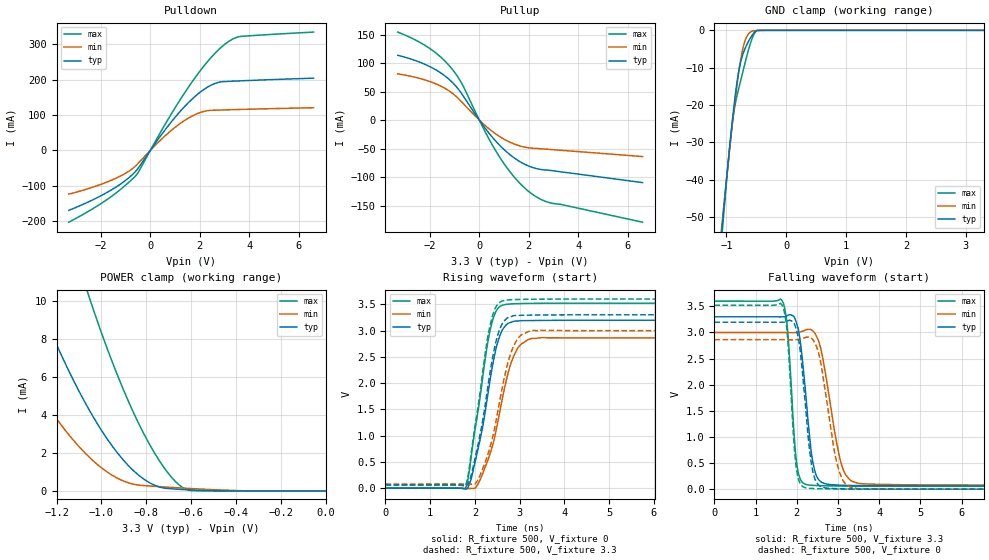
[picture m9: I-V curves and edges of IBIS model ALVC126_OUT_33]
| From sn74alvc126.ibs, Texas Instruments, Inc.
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[Model]   ALVC126_OUT_33
Model_type  3-state
Enable   Active-High
Vref =   0
Rref =   500
Cref =   50p
Vmeas =   1.5
| variable   typ   min   max
C_comp   4.92pF   4.23pF   5.84pF
| C_pullup   6.06pF   4.27pF   7.77pF
| C_pulldown   7.87pF   4.86pF   12.41pF
| C_tri-state   4.92pF   4.23pF   5.84pF
[Temperature Range]   40   100   -40
| Ambient temperature   25   85   -40
[Voltage range]   3.3   3   3.6
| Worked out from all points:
|   slope of the pulldown table from 0 to 0.495 V, typ, clamps not added: 10.2 ohm
|   slope of the pullup table from 0 to 0.495 V, typ, clamps not added: 17.4 ohm
|   GND clamp passes 1 mA (typ) near -0.56 V on its own axis
|   POWER clamp passes 1 mA (typ) near -0.85 V on its own axis
|   rising waveform, R_fixture 500, V_fixture 0: 20-80 % time 405ps typ, 469ps min, 364ps max; typ from 0 V to 3.2 V
|   falling waveform, R_fixture 500, V_fixture 3.3: 20-80 % time 240ps typ, 374ps min, 169ps max; typ from 3.3 V to 0.064 V
|   rising waveform, R_fixture 500, V_fixture 3.3: 20-80 % time 395ps typ, 450ps min, 358ps max; typ from 0.064 V to 3.3 V
|   falling waveform, R_fixture 500, V_fixture 0: 20-80 % time 232ps typ, 343ps min, 164ps max; typ from 3.2 V to 0 V
[GND Clamp]
| ALVC126_OUT_33
|   Voltage   I(typ)   I(min)   I(max)
-3.3V     -502.3mA   -462.6mA   -544.6mA
-1.08V    -54.25mA   -52.87mA   -55.93mA
-1.06V    -50.69mA   -49.62mA   -52.05mA
-965mV    -34.4mA    -34.63mA   -34.59mA
-900mV    -24.12mA   -24.99mA   -24.7mA
-860mV    -18.44mA   -19.43mA   -20.39mA
-805mV    -11.98mA   -12.5mA    -16.29mA
-705mV    -5.559mA   -3.602mA   -9.787mA
-655mV    -3.719mA   -1.531mA   -6.626mA
-575mV    -1.408mA   -240.7uA   -2.39mA
-480mV    -21.04uA   -62.18uA   -16.51uA
3.3V      104.8pA    1.494uA    43.91pA
[POWER Clamp]
| ALVC126_OUT_33
|   Voltage   I(typ)   I(min)   I(max)
-3.3V     101.4mA    70.85mA    144.9mA
-1.515V   17.49mA    10.21mA    30.43mA
-1.39V    13.28mA    7.381mA    24.27mA
-1.295V   10.36mA    5.473mA    19.9mA
-1.175V   7.064mA    3.406mA    14.79mA
-1.055V   4.279mA    1.788mA    10.22mA
-950mV    2.335mA    812.2uA    6.743mA
-845mV    938.6uA    325.5uA    3.823mA
-745mV    219.5uA    228.1uA    1.65mA
-655mV    86.61uA    162.8uA    329uA
-600mV    50.74uA    125.6uA    17.36uA
-48.03fV  104.8pA    414.1pA    48.4pA
[Pulldown]
| ALVC126_OUT_33
|   Voltage   I(typ)   I(min)   I(max)
-3.3V     -169.5mA   -123.9mA   -203mA
-1.625V   -113.8mA   -85.92mA   -132.9mA
-1.02V    -85.87mA   -65.43mA   -99.42mA
-590mV    -58.76mA   -43.67mA   -71.86mA
600mV     58.25mA    41.24mA    73.83mA
1.525V    133.8mA    90.44mA    177mA
2.34V     179.7mA    112.3mA    253mA
2.695V    190.8mA    113.5mA    279.9mA
3.025V    194.3mA    114.3mA    300.3mA
3.355V    195.4mA    114.9mA    315.1mA
3.65V     196.3mA    115.5mA    321.7mA
6.6V      203.8mA    120.3mA    334mA
[Pullup]
| ALVC126_OUT_33
|   Voltage   I(typ)   I(min)   I(max)
-3.3V     113.7mA    81.1mA     154.3mA
-2.045V   94.71mA    68.29mA    126.7mA
-1.555V   82.58mA    59.54mA    110.3mA
-1.135V   67.94mA    48.5mA     91.26mA
-685mV    44.37mA    30.46mA    62.31mA
200mV     -12.17mA   -8.178mA   -17.55mA
785mV     -42.51mA   -27.85mA   -62.43mA
1.415V    -66.5mA    -42.01mA   -100.1mA
2.045V    -81.49mA   -48.91mA   -126.8mA
2.445V    -86.35mA   -50.12mA   -138.1mA
2.85V     -88.18mA   -51.47mA   -145mA
6.6V      -109.6mA   -63.97mA   -179.1mA
[Ramp]
| ALVC126_OUT_33
| variable   typ   min   max
dV/dt_r   1.93/4.10E-10   1.72/4.78E-10   2.12/3.68E-10
dV/dt_f   1.97/2.53E-10   1.79/3.89E-10   2.15/1.78E-10
R_load = 500
[Rising Waveform]
| ALVC126_OUT_33
R_fixture =   500
C_fixture =   0
L_fixture =   0
V_fixture =   0
V_fixture_min = 0
V_fixture_max = 0
|   Time   V(typ)   V(min)   V(max)
0s        33.51pV    1.907nV    27.94pV
1.78ns    -11.41mV   -1.75mV    -14.61mV
1.945ns   280.2mV    -4.234mV   783.1mV
2.18ns    1.202V     293.1mV    2.158V
2.35ns    2.124V     689.7mV    3.048V
2.53ns    2.838V     1.345V     3.438V
2.725ns   3.128V     2.139V     3.503V
3.01ns    3.187V     2.724V     3.514V
3.52ns    3.194V     2.866V     3.52V
50ns      3.197V     2.862V     3.521V
[Falling Waveform]
| ALVC126_OUT_33
R_fixture =   500
C_fixture =   0
L_fixture =   0
V_fixture =   3.3
V_fixture_min = 3
V_fixture_max = 3.6
|   Time   V(typ)   V(min)   V(max)
0s        3.3V       3V         3.6V
1.655ns   3.3V       3V         3.592V
1.775ns   3.324V     2.999V     3.055V
2.005ns   3.154V     3V         452.2mV
2.12ns    2.596V     3.02V      147.2mV
2.33ns    863.9mV    3.058V     75.48mV
2.585ns   140mV      2.683V     67.18mV
3.11ns    74.4mV     410.1mV    58.46mV
3.645ns   66.34mV    100.5mV    56.19mV
50ns      63.7mV     79.91mV    56.01mV
[Rising Waveform]
| ALVC126_OUT_33
R_fixture =   500
C_fixture =   0
L_fixture =   0
V_fixture =   3.3
V_fixture_min = 3
V_fixture_max = 3.6
|   Time   V(typ)   V(min)   V(max)
0s        63.7mV     79.91mV    56.01mV
1.78ns    52.24mV    77.86mV    41.44mV
1.86ns    108.8mV    74.8mV     311.8mV
2ns       561.6mV    79.22mV    1.179V
2.34ns    2.221V     791.9mV    3.108V
2.52ns    2.945V     1.504V     3.514V
2.72ns    3.238V     2.334V     3.582V
3.005ns   3.291V     2.894V     3.593V
3.515ns   3.297V     3.006V     3.599V
50ns      3.3V       3V         3.6V
[Falling Waveform]
| ALVC126_OUT_33
R_fixture =   500
C_fixture =   0
L_fixture =   0
V_fixture =   0
V_fixture_min = 0
V_fixture_max = 0
|   Time   V(typ)   V(min)   V(max)
0s        3.197V     2.862V     3.521V
1.65ns    3.197V     2.862V     3.512V
1.765ns   3.216V     2.861V     3.01V
1.99ns    3.054V     2.862V     395.2mV
2.1ns     2.528V     2.877V     83.95mV
2.315ns   720.7mV    2.908V     14.36mV
2.555ns   64.51mV    2.52V      8.765mV
3.025ns   8.013mV    356mV      2.361mV
3.485ns   2.48mV     11.05mV    329uV
50ns      -6.58nV    6.337nV    -6.738nV
